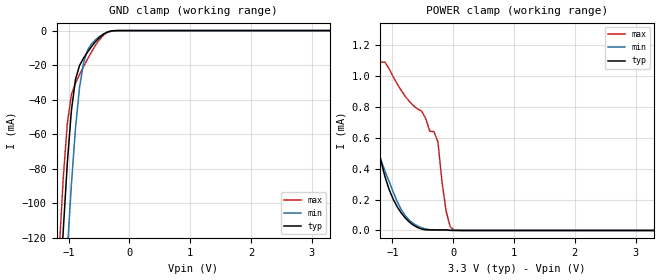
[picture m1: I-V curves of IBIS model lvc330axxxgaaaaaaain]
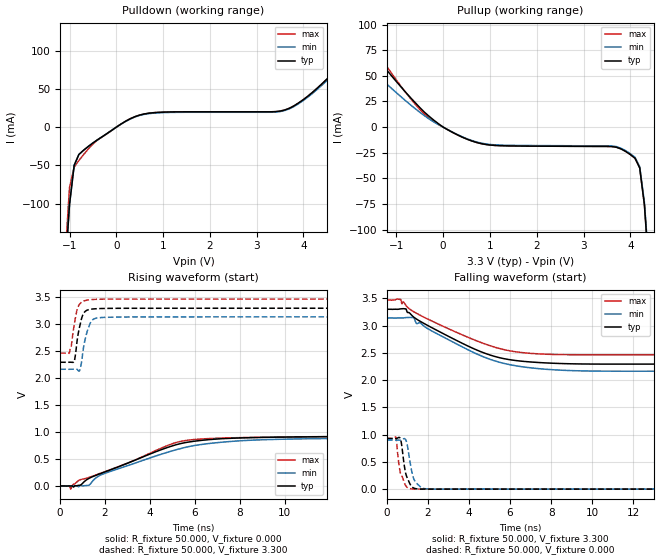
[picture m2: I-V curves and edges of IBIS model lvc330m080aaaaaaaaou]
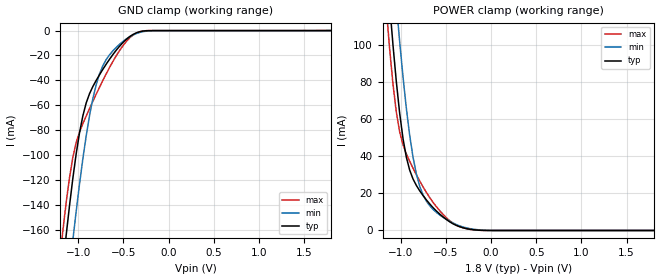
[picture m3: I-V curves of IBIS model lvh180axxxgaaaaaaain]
| IBIS Models Generator: Lattice Radiant Software (64-bit) 2023.2.1.288.0
| Report Generate Date: Aug 26 2024
| Report Generate Time: 15:07:20
| IBIS File LibisMaker.ibs
| Cadence Design Systems, Inc. 2022
[IBIS ver]   4.2
[File Name]   LAB05_impl_1.ibs
[File Rev]   1.8
[Date]   Mon Jul 10 07:12:10 PDT 2023
[Source]   Lattice Semiconductor 28fdsoi Process
[Notes]   Device: LFCPNX-100   Final
   Lattice Semiconductor has worked hard to ensure the
   models below are accurate and complete.  However, the
   data below was generated using simulation of the
   input/output model files for the silicon.  Therefore,
   the data below is for reference and initial design
   purposes only.
   Lattice Semiconductor grants permission to use this
   data for use in printed circuit design using this
   Lattice programmable logic device.  Other use of this
   code, including the selling or duplication of any
   portion is strictly prohibited.
|   NAMING CONVENTION
   The IBIS [Model] header is limited by the specification to a
   total of characters.  With such a set of characters available
   for naming models it becomes important to attempt to
   meaningfully encode the IO standards so they fit within the
   twenty character limit.  It would seem that twenty characters
   would provide room enough for describing IO's.  However, the
   PLD IO structure continues to grow more and more complex.  The
   complexity is making the twenty characters insuffiently
   descriptive.  In order to overcome this issue the naming
   convention described below is implemented to resolve the issue.
The twenty character space is managed as follows:
   bbbvvvsdddprttmaoixx
   b = standard
   v = voltage (x.xx V)
   s = slew code
   d = drive (xx.x ma)
   p = pullmode code
   r = impedance
   t = termination code
   m = mipi hard dphy mode
   o = diff resistor code
   i = diff  current code
   x = reserved
   standard
   LVCMOS   lvc
   LVCMOSH   lvh
   LVCMOSR   lvr
   LVCMOSD   lvd
   LVTTL   lvt
   lvttld   ltd
   sstl_I   ss1
   sstl_II   ss2
   sstld_I   s1d
   sstld_II   s2d
   hsul   hs1
   hsuld   h1d
   hstl_I   hs1
   hstld_I   h1d
   lvds   lvs
   lvdse   lve
   SUBLVDS   slv
   sublvdse   sle
   sublvdseh   slh
   slvs   svs
   mipi   mip
   vref1   vr1
   lvstl_I   ll1
   lvstl_II   ll2
   lvstld_I   l1d
   lvstld_II   l2d
   slew
   na   a
   fast   f
   slow   s
   med   m
   drive
   2   020
   4   040
   6   060
   8   080
   10   100
   12   120
   16   160
   50rs   r50
   na   xxx
   pullmode/clamp on
   none   a/e
   failsafe   a/e
   up   b/f
   down   c/g
   keeper   d/h
   i3c   i
   impedance
   off   a
   termination
   off   aa
   40   bb
   50   cc
   60   dd
   75   ee
   150   ff
   48   gg
   80   hh
   120   ii
   mipi hard dphy mode
   off   a
   lp   l
   hs   h
   differential resistor
   off   a
   100   b
   differential current
   NA   a
   2.0   b
   3.5   c
   Reserved   IO type
   in   input only (mipi: rx)
   ou   output (mipi: tx)
   io   I/O
   od   Open drain
   ic   Inverting differential input
  (signal name only)
   it   Non-Inverting differential
  input (signal name only)
   on   Inverting differential output
  (signal name only)
   op   Non-Inverting differential
  output (signal name only)
   All the IO models are generated with pull mode set to none.
   Lattice Semiconductor Corporation
   5555 NE Moore Court
   Hillsboro, OR 97214
   U.S.A
   TEL: 1-800-Lattice (USA and Canada)
   408-826-6000 (other locations)
   web: http://www.latticesemi.com/
   email: techsupport@latticesemi.com
[Disclaimer] This IBIS source code is intended as a design reference
   which illustrates how the Lattice Semiconductor device operates.
   It is the user's responsibility to verify their design for
   consistency and functionality through the use of formal
   verification methods.  Lattice Semiconductor provides no warranty
   regarding the use or functionality of this data.
[Copyright]   Copyright 2022 by Lattice Semiconductor Corporation
|   Component LFCPNX
[Component] LFCPNX
[Manufacturer] Lattice Semiconductor Corp.
[Package]
|LFG672
| variable   typ   min   max
R_pkg   0.85482   0.28979   1.626
L_pkg   4.948e-9   1.752e-9   8.572e-9
C_pkg   1.721e-12   9.177e-13   2.607e-12
[Pin]  signal_name   model_name   R_pin   L_pin   C_pin
AE26   Digit_en[2]   lvh180m080eaaaaaaaou
W22   Digit_en[1]   lvh180m080eaaaaaaaou
AC21   Digit_en[0]   lvh180m080eaaaaaaaou
M4   seg_out[6]   lvc330m080aaaaaaaaou
M3   seg_out[5]   lvc330m080aaaaaaaaou
M2   seg_out[4]   lvc330m080aaaaaaaaou
M1   seg_out[3]   lvc330m080aaaaaaaaou
N1   seg_out[2]   lvc330m080aaaaaaaaou
N2   seg_out[1]   lvc330m080aaaaaaaaou
N3   seg_out[0]   lvc330m080aaaaaaaaou
AA23   Dir   lvh180axxxgaaaaaaain
N9   rst_n   lvc330axxxgaaaaaaain
| Models and submodels in the file (4): lvc330axxxgaaaaaaain (Input), lvc330m080aaaaaaaaou (Output), lvh180axxxgaaaaaaain (Input), lvh180m080eaaaaaaaou (Output)
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[Model] lvc330axxxgaaaaaaain
Model_type Input
Polarity   Non-Inverting
Enable   Active-High
Vinl =  0.800V
Vinh =  2.000V
C_comp   5.000pF   4.000pF   5.500pF
[Temperature Range]   25.000   0.125k   -40.000
[Voltage Range]   3.300V   3.140V   3.470V
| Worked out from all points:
|   GND clamp passes 1 mA (typ) near -0.37 V on its own axis
|   POWER clamp passes 1 mA (typ) near -1.47 V on its own axis
[GND_clamp]
|Voltage   I(typ)   I(min)   I(max)
-3.3V     -1.865A    -1.847A    -1.883A
-1.156V   -160.1mA   -214.1mA   -127.6mA
-1.089V   -115.7mA   -169.6mA   -85.35mA
-1.022V   -76.45mA   -127.5mA   -53.7mA
-955mV    -46.24mA   -89.13mA   -37.05mA
-888mV    -28.3mA    -56.66mA   -30.41mA
-821mV    -20.19mA   -32.82mA   -25.49mA
-754mV    -15.89mA   -18.49mA   -20.81mA
-620mV    -9.094mA   -7.515mA   -12.09mA
-419mV    -1.868mA   -1.846mA   -2.383mA
-218mV    -16.48uA   -78.61uA   -6.639uA
3.3V      0A         0A         0A
[POWER_clamp]
|Voltage   I(typ)   I(min)   I(max)
-3.3V     37.53mA    9.364mA    73.7mA
-1.792V   1.823mA    1.318mA    2.466mA
-1.591V   1.29mA     991.8uA    1.714mA
-1.457V   981.8uA    795.4uA    1.299mA
-1.39V    843.7uA    703.6uA    1.091mA
-1.122V   347.7uA    385.2uA    1.091mA
-854mV    112.9uA    134.5uA    907uA
-586mV    19.15uA    28.85uA    788.2uA
-251mV    3.861uA    1.254uA    573.3uA
-117mV    3.861uA    1.254uA    126.7uA
17mV      69.96nA    1.254uA    1.636uA
3.3V      0A         0A         0A
[Model] lvc330m080aaaaaaaaou
Model_type Output
Polarity   Non-Inverting
Enable   Active-High
Vmeas =  1.650V
Cref =  0.0F
Rref =  1.000M
Vref =  0.0V
C_comp   5.000pF   4.000pF   5.500pF
[Temperature Range]   25.000   0.125k   -40.000
[Voltage Range]   3.300V   3.140V   3.470V
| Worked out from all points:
|   slope of the pulldown table from 0 to 0.495 V, typ, clamps not added: 31.5 ohm
|   slope of the pullup table from 0 to 0.495 V, typ, clamps not added: 43.2 ohm
|   rising waveform, R_fixture 50.000, V_fixture 0.000: 20-80 % time 3.47ns typ, 3.91ns min, 3.27ns max; typ from 0 V to 0.929 V
|   rising waveform, R_fixture 50.000, V_fixture 3.300: 20-80 % time 248ps typ, 295ps min, 236ps max; typ from 2.3 V to 3.3 V
|   falling waveform, R_fixture 50.000, V_fixture 3.300: 20-80 % time 3.22ns typ, 3.2ns min, 3.51ns max; typ from 3.3 V to 2.3 V
|   falling waveform, R_fixture 50.000, V_fixture 0.000: 20-80 % time 273ps typ, 284ps min, 288ps max; typ from 0.929 V to 0 V
[Pulldown]
|Voltage   I(typ)   I(min)   I(max)
-3.3V     -3.025A    -3.025A    -3.918A
-1.1V     -192.9mA   -192.9mA   -175.3mA
-1V       -101.2mA   -101.2mA   -78.95mA
-900mV    -49.86mA   -49.86mA   -52.21mA
-800mV    -35.81mA   -35.81mA   -43.74mA
200mV     7.775mA    7.542mA    7.775mA
800mV     18.91mA    18.34mA    18.91mA
3.6V      22.45mA    21.77mA    22.45mA
4.1V      40.8mA     39.58mA    40.8mA
5.4V      113.7mA    110.3mA    113.7mA
6.1V      131.6mA    127.7mA    131.6mA
6.6V      184.5mA    179mA      184.5mA
[Pullup]
|Voltage   I(typ)   I(min)   I(max)
-3.3V     145.5mA    90.7mA     185.8mA
-2.7V     96.8mA     74.7mA     125.4mA
-2.1V     95.1mA     70.11mA    105.4mA
-1.8V     86.3mA     64.15mA    96.9mA
-500mV    19.13mA    14.57mA    17.21mA
0V        28.62nA    228.6nA    28.62nA
600mV     -13.29mA   -12.89mA   -13.29mA
3.9V      -23.67mA   -22.96mA   -23.67mA
4.2V      -39.73mA   -38.54mA   -39.73mA
4.3V      -75.4mA    -73.1mA    -75.4mA
4.4V      -140.5mA   -136.3mA   -140.5mA
6.6V      -2.178A    -2.113A    -2.178A
[Ramp]
| variable   typ   min   max
dV/dt_r   0.789/3.474n   0.590/3.936n   0.521/3.276n
dV/dt_f   0.706/3.253n   0.547/3.212n   0.513/3.516n
R_load = 50.000
[Rising Waveform]
R_fixture = 50.000
V_fixture = 0.000
V_fixture_min = 0.000
V_fixture_max = 0.000
|  time   V(typ)   V(min)   V(max)
0s        488.9uV    1.198mV    488.9uV
395ps     637.6uV    952.2uV    3.238mV
475ps     718.1uV    1.204mV    -58.62mV
816ps     11.39mV    -13.02mV   99.9mV
1.256ns   135.1mV    11.8mV     155.5mV
2.016ns   265mV      239.2mV    270.5mV
4.885ns   729.4mV    638.7mV    767.7mV
5.78ns    819.5mV    735.4mV    854.8mV
9.109ns   902.9mV    859.8mV    905.4mV
20ns      929.1mV    899.7mV    931mV
[Rising Waveform]
R_fixture = 50.000
V_fixture = 3.300
V_fixture_min = 3.140
V_fixture_max = 3.470
|  time   V(typ)   V(min)   V(max)
0s        2.297V     2.167V     2.467V
409ps     2.297V     2.166V     2.466V
616ps     2.299V     2.168V     2.961V
734ps     2.622V     2.168V     3.237V
866ps     2.953V     2.141V     3.375V
1.036ns   3.197V     2.555V     3.43V
1.276ns   3.274V     2.953V     3.455V
1.486ns   3.287V     3.096V     3.463V
2.077ns   3.297V     3.131V     3.469V
20ns      3.3V       3.14V      3.47V
[Falling Waveform]
R_fixture = 50.000
V_fixture = 3.300
V_fixture_min = 3.140
V_fixture_max = 3.470
|  time   V(typ)   V(min)   V(max)
0s        3.3V       3.14V      3.47V
666ps     3.307V     3.141V     3.481V
726ps     3.309V     3.14V      3.403V
924ps     3.306V     3.147V     3.369V
1.275ns   3.165V     3.146V     3.261V
1.436ns   3.12V      3.04V      3.227V
4.236ns   2.575V     2.505V     2.741V
6.39ns    2.354V     2.256V     2.514V
9.897ns   2.295V     2.167V     2.465V
20ns      2.297V     2.167V     2.467V
[Falling Waveform]
R_fixture = 50.000
V_fixture = 0.000
V_fixture_min = 0.000
V_fixture_max = 0.000
|  time   V(typ)   V(min)   V(max)
0s        929.1mV    899.7mV    931mV
432ps     928.7mV    899.2mV    951mV
635ps     935.9mV    899.2mV    328.3mV
704ps     834.8mV    904.4mV    247.5mV
846ps     423.4mV    926.9mV    115mV
936ps     256.3mV    884.1mV    51.1mV
1.193ns   51.59mV    350.2mV    4.707mV
1.432ns   6.847mV    110.5mV    217.4uV
1.966ns   398.9uV    3.886mV    -527.1uV
20ns      488.9uV    1.198mV    488.9uV
[Model] lvh180axxxgaaaaaaain
Model_type Input
Polarity   Non-Inverting
Enable   Active-High
Vinl =  0.630V
Vinh =  1.170V
C_comp   5.000pF   4.000pF   5.500pF
[Temperature Range]   25.000   0.125k   -40.000
[Voltage Range]   1.800V   1.710V   1.890V
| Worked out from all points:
|   GND clamp passes 1 mA (typ) near -0.32 V on its own axis
|   POWER clamp passes 1 mA (typ) near -0.27 V on its own axis
[GND_clamp]
|Voltage   I(typ)   I(min)   I(max)
-1.8V     -677.5mA   -713mA     -658.3mA
-1.171V   -189.9mA   -242.9mA   -161.4mA
-1.134V   -164.8mA   -217.4mA   -138.4mA
-1.06V    -118.9mA   -168.5mA   -102mA
-1.023V   -99.16mA   -145.4mA   -89.98mA
-949mV    -68.55mA   -103.1mA   -74.79mA
-838mV    -44.93mA   -54.66mA   -56.82mA
-764mV    -35.44mA   -34.74mA   -45.46mA
-616mV    -19.23mA   -16.23mA   -24.76mA
-394mV    -3.128mA   -3.569mA   -3.61mA
-246mV    -140.7uA   -457.2uA   -76.91uA
1.8V      0A         0A         0A
[POWER_clamp]
|Voltage   I(typ)   I(min)   I(max)
-1.8V     630.7mA    657.6mA    617.2mA
-1.16V    145.7mA    191.9mA    120mA
-1.123V   122.1mA    167.9mA    98mA
-1.086V   100.1mA    144.7mA    78.99mA
-1.049V   80.33mA    122.6mA    63.89mA
-1.012V   63.31mA    101.9mA    53.2mA
-938mV    39.5mA     65.89mA    41.31mA
-864mV    27.77mA    39.53mA    33.58mA
-790mV    21.38mA    23.82mA    26.71mA
-457mV    4.636mA    4.921mA    5.201mA
-124mV    126.2uA    290uA      82.78uA
1.8V      0A         0A         0A
